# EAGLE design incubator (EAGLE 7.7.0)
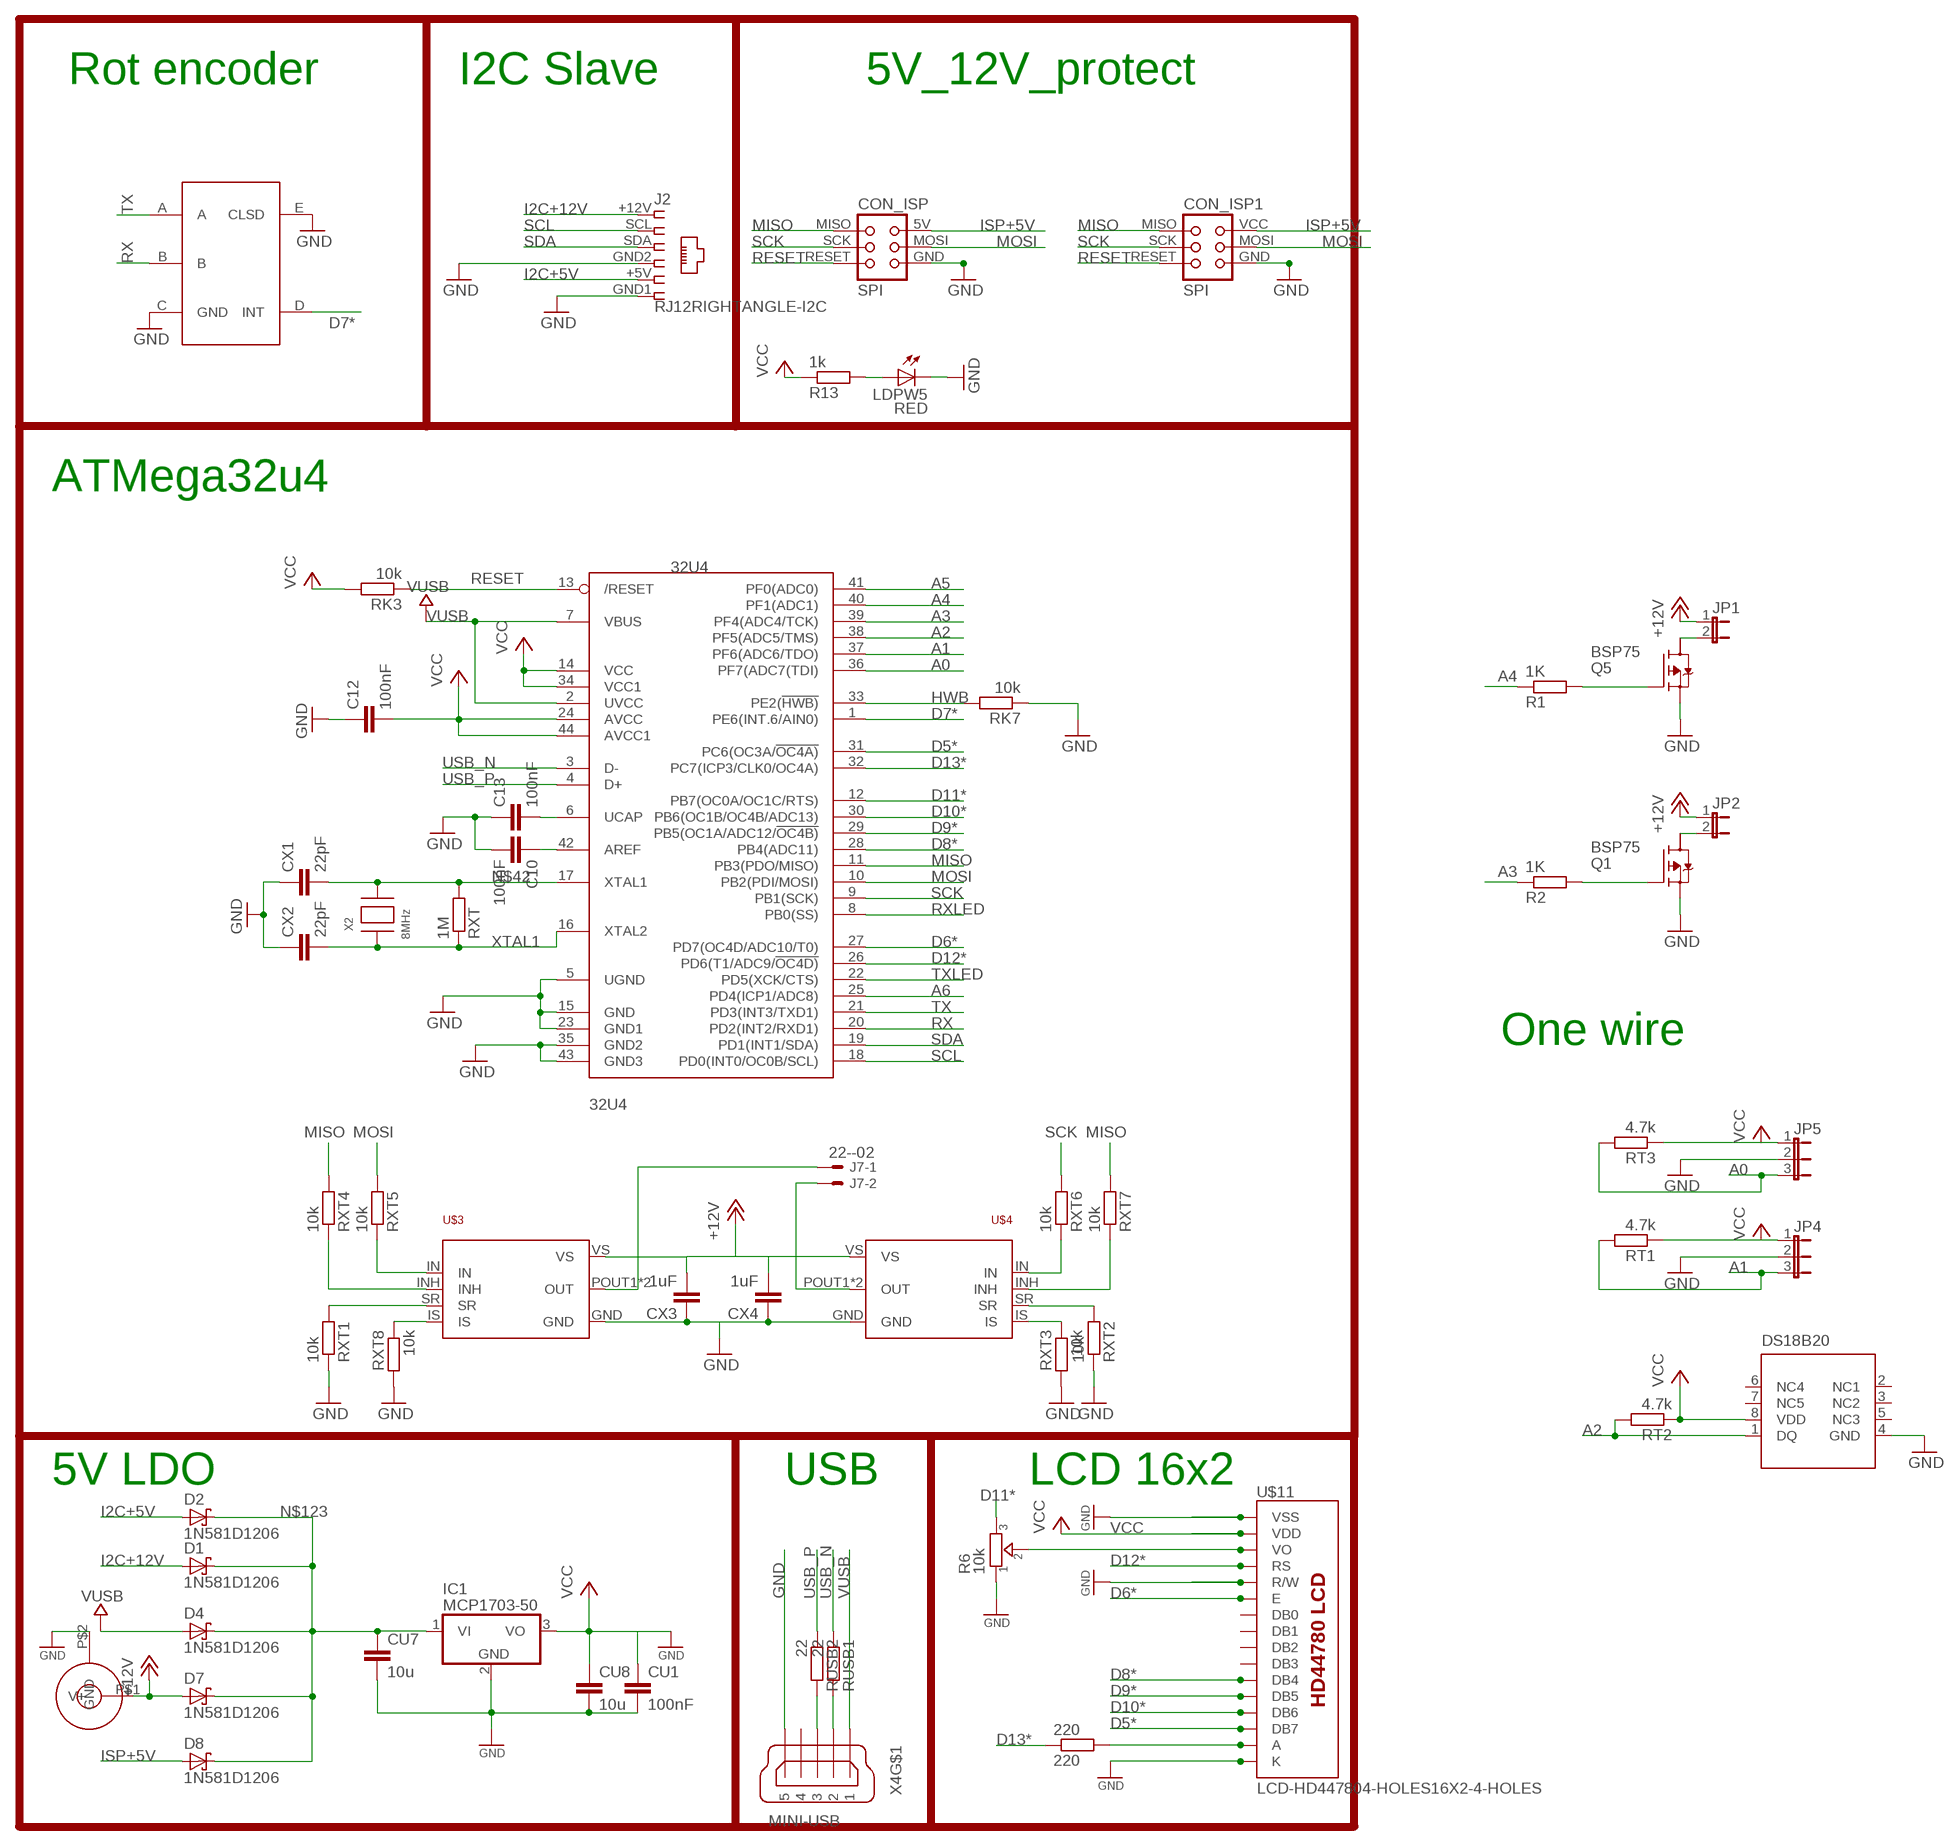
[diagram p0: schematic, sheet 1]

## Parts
32U4  32U4  ATMEGA32U4-AU  [TQFP44]
220  220  R-EU_R0805  [R0805]
C10  100nF  C-EUC0805  [C0805]
C12  100nF  C-EUC0805  [C0805]
C13  100nF  C-EUC0805  [C0805]
CON_ISP  SPI  TINYISPT  [TC2030-MCP-NL]
CON_ISP1  SPI  TINYISP  [TINYISP]
CU1  100nF  C-EUC0805  [C0805]
CU7  10u  C-EUC0805  [C0805]
CU8  10u  C-EUC0805  [C0805]
CX1  22pF  C-EUC0805  [C0805]
CX2  22pF  C-EUC0805  [C0805]
CX3  1uF  C-EUC0805  [C0805]
CX4  1uF  C-EUC0805  [C0805]
D1  1N581D1206  [LED-1206]
D2  1N581D1206  [LED-1206]
D4  1N581D1206  [LED-1206]
D7  1N581D1206  [LED-1206]
D8  1N581D1206  [LED-1206]
IC1  MCP1703-50  MCP1703DB  [SOT223]
J2  RJ12RIGHTANGLE-I2C  [RJ12-RIGHTANGLE-I2C]
J7  22--02  [2-PIN-5.08S]
JP1  JUMPER-2PTH  [1X02]
JP2  JUMPER-2PTH  [1X02]
JP4  JP2E  [JP2]
JP5  JP2E  [JP2]
LDPW5  RED  LEDCHIP-LED0805  [CHIP-LED0805]
POWER  JACK_DC_BARREL  [DC_BARREL]
Q1  BSP75  BSP613P  [PG-SOT-223]
Q5  BSP75  BSP613P  [PG-SOT-223]
R1  1K  R-EU_R0805  [R0805]
R2  1K  R-EU_R0805  [R0805]
R6  10k  TRIMMER-3362P  [TRIMMER_3362P]
R13  1k  R-EU_R0805  [R0805]
RK3  10k  R-EU_M0805  [M0805]
RK7  10k  R-EU_M0805  [M0805]
RT1  4.7k  R-EU_R0805  [R0805]
RT2  4.7k  R-EU_R0805  [R0805]
RT3  4.7k  R-EU_R0805  [R0805]
RUSB1  22  R-EU_M0805  [M0805]
RUSB2  22  R-EU_M0805  [M0805]
RXT  1M  R-EU_R0805  [R0805]
RXT1  10k  R-EU_R0805  [R0805]
RXT2  10k  R-EU_R0805  [R0805]
RXT3  10k  R-EU_R0805  [R0805]
RXT4  10k  R-EU_R0805  [R0805]
RXT5  10k  R-EU_R0805  [R0805]
RXT6  10k  R-EU_R0805  [R0805]
RXT7  10k  R-EU_R0805  [R0805]
RXT8  10k  R-EU_R0805  [R0805]
U$1  EC11E  [EC11E]
U$3  BTS7960  [P-TO-263-7]
U$4  BTS7960  [P-TO-263-7]
U$5  DS18B20  DS18B20SMALL  [MSOP8]
U$11  LCD-HD447804-HOLES16X2-4-HOLES  [LCD-16X2-4HOLES]
X2  8MHz  XTALNX6035  [NX6035]
X4  MINI-USB  MINI-USB-SCHIELD-32005-201  [32005-201]

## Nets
+12V [power]: CX3.2 CX4.2 D7.A JP1.1 JP2.1 POWER.P$1(V+) U$3.VS U$4.VS
A0: 32U4.36(PF7(ADC7(TDI)) JP5.3 RT3.2
A1: 32U4.37(PF6(ADC6/TDO)) JP4.3 RT1.2
A2: 32U4.38(PF5(ADC5/TMS)) RT2.2 U$5.1(DQ)
A3: 32U4.39(PF4(ADC4/TCK)) R2.1
A4: 32U4.40(PF1(ADC1)) R1.1
A5: 32U4.41(PF0(ADC0))
A6: 32U4.25(PD4(ICP1/ADC8))
AREF: 32U4.42(AREF) C10.1
D5*: 32U4.31(PC6(OC3A/!OC4A)) U$11.14(DB7)
D6*: 32U4.27(PD7(OC4D/ADC10/T0)) U$11.6(E)
D7*: 32U4.1(PE6(INT.6/AIN0)) U$1.D(INT)
D8*: 32U4.28(PB4(ADC11)) U$11.11(DB4)
D9*: 32U4.29(PB5(OC1A/ADC12/!OC4B)) U$11.12(DB5)
D10*: 32U4.30(PB6(OC1B/OC4B/ADC13)) U$11.13(DB6)
D11*: 32U4.12(PB7(OC0A/OC1C/RTS)) R6.3
D12*: 32U4.26(PD6(T1/ADC9/!OC4D)) U$11.4(RS)
D13*: 32U4.32(PC7(ICP3/CLK0/OC4A)) 220.1
GND [power]: 32U4.5(UGND) 32U4.15(GND) 32U4.23(GND1) 32U4.35(GND2) 32U4.43(GND3) C10.2 C12.1 C13.1 CON_ISP1.GND CON_ISP.GND CU1.2 CU7.2 CU8.2 CX1.1 CX2.1 CX3.1 CX4.1 IC1.2(GND) J2.GND1 J2.GND2 JP4.2 JP5.2 LDPW5.C POWER.P$2(GND) Q1.3(S) Q5.3(S) R6.1 RK7.1 RXT1.1 RXT2.1 RXT3.2 RXT8.2 U$1.C(GND) U$1.E(CLSD) U$3.GND U$4.GND U$5.4(GND) U$11.1(VSS) U$11.5(R/W) U$11.16(K) X4.5
HWB: 32U4.33(PE2(!HWB)) RK7.2
I2C+5V: D2.A J2.+5V
I2C+12V [power]: D1.A J2.+12V
ISP+5V: CON_ISP1.VCC CON_ISP.5V(VCC) D8.A
MISO: 32U4.11(PB3(PDO/MISO)) CON_ISP1.MISO CON_ISP.MISO RXT4.2 RXT7.2
MOSI: 32U4.10(PB2(PDI/MOSI)) CON_ISP1.MOSI CON_ISP.MOSI RXT5.2
N$1: 32U4.6(UCAP) C13.2
N$2: R6.2 U$11.3(VO)
N$4: RXT5.1 U$3.IN
N$5: RXT6.1 U$4.IN
N$6: RXT4.1 U$3.INH
N$7: RXT7.1 U$4.INH
N$8: RXT3.1 U$4.IS
N$9: Q5.1(G) R1.2
N$10: RXT2.2 U$4.SR
N$11: 220.2 U$11.15(A)
N$12: LDPW5.A R13.2
N$13: RXT1.2 U$3.SR
N$14: RXT8.1 U$3.IS
N$19: J7.1 U$3.POUT1(OUT) U$3.POUT2(OUT)
N$20: Q1.1(G) R2.2
N$21: JP1.2 Q5.2(D)
N$22: J7.2 U$4.POUT1(OUT) U$4.POUT2(OUT)
N$23: JP2.2 Q1.2(D)
N$42: 32U4.17(XTAL1) CX1.2 RXT.2 X2.P$2
N$123: CU7.1 D1.C D2.C D4.C D7.C D8.C IC1.1(VI)
RESET: 32U4.13(/RESET) CON_ISP1.RESET CON_ISP.RESET RK3.1
RX: 32U4.20(PD2(INT2/RXD1)) U$1.B
RXLED: 32U4.8(PB0(SS))
SCK: 32U4.9(PB1(SCK)) CON_ISP1.SCK CON_ISP.SCK RXT6.2
SCL: 32U4.18(PD0(INT0/OC0B/SCL)) J2.SCL
SDA: 32U4.19(PD1(INT1/SDA)) J2.SDA
TX: 32U4.21(PD3(INT3/TXD1)) U$1.A
TXLED: 32U4.22(PD5(XCK/CTS))
USB_N: 32U4.3(D-) RUSB1.1
USB_P: 32U4.4(D+) RUSB2.1
USBC_N: RUSB1.2 X4.2
USBC_P: RUSB2.2 X4.3
VCC: 32U4.14(VCC) 32U4.24(AVCC) 32U4.34(VCC1) 32U4.44(AVCC1) C12.2 CU1.1 CU8.1 IC1.3(VO) JP4.1 JP5.1 R13.1 RK3.2 RT1.1 RT2.1 RT3.1 U$5.8(VDD) U$11.2(VDD) ; supply symbol labelled GND
VUSB: 32U4.2(UVCC) 32U4.7(VBUS) D4.A X4.1
XTAL1: 32U4.16(XTAL2) CX2.2 RXT.1 X2.P$1
Unconnected: Q1.4(D) Q5.4(D) U$5.2(NC1) U$5.3(NC2) U$5.5(NC3) U$5.6(NC4) U$5.7(NC5) U$11.7(DB0) U$11.8(DB1) U$11.9(DB2) U$11.10(DB3) X4.4 X4.M1(S:S1) X4.M2(S:S2) X4.M3(S:S3) X4.M4(S:S4)

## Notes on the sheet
- Rot encoder | I2C Slave | 5V_12V_protect
- ATMega32u4
- One wire
- 5V LDO | USB | LCD 16x2

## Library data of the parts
32U4 = adafruit:ATMEGA32U4: http://www.ladyada.net/library/eagle
220 R1 R2 RXT RXT1-RXT8 = rcl:R-EU_: RESISTOR, European symbol
C10 C12 C13 CU1 CU7 CU8 CX1-CX4 = rcl:C-EU: CAPACITOR, European symbol
CON_ISP = lpatiny:TINYISP: CONNECTOR
CON_ISP1 = lpatiny:TINYISP: CONNECTOR; OC_FARNELL: unknown; OC_NEWARK: unknown
D1 D2 D4 D7 D8 = lpatiny:1N581*: 1.0A SCHOTTKY BARRIER RECTIFIER
IC1 = linear:MCP1703: 250 mA, 16V, Low Quiescent Current LDO Regulator Source: http://ww1.microchip.com/downloads/en/DeviceDoc/22049b.pdf
J2 = lpatiny:RJ12: CORCOM Modular RJ Jacks No Shield Source: www.tycoelectronics.com .. ENG_DS_1654001_1099_RJ_L_0507.pdf
J7 = lpatiny:22-?-02: CONNECTOR
JP1 JP2 = SparkFun:JUMPER-2: Jumper
JP4 JP5 = jumper:JP2E: JUMPER
LDPW5 = adafruit:LED: LED
POWER = lpatiny:JACK_DC_BARREL
Q1 Q5 = infineon:BSP613P: SIPMOS (R) Small-Signal-Transistor P-Channel (2 Drain) Source: http://www.infineon.com/dgdl/BSP613P_Rev2.4.pdf; OC_FARNELL: unknown; OC_NEWARK: unknown
R6 = dp_devices:TRIMMER: Trimmer resistor
R13 RK3 RK7 RT1-RT3 RUSB1 RUSB2 = resistor:R-EU_: RESISTOR, European symbol
U$1 = lpatiny:EC11E: ALPS Rotary encoder
U$3 U$4 = BTS7960:BTS7960; AVAILABILITY: Warning; DESCRIPTION: Half Bridge Motor Driver 7-Pin%286%2BTab%29 TO-263; MF: Infineon; MP: BTS7960B; PACKAGE: TO-263 Infineon; PRICE: 4.95 USD
U$5 = lpatiny:DS18B20
U$11 = HD44780LCD:LCD-HD44780
X2 = lpatiny:XTAL: Low cost SMT crystals, no capacitors included
X4 = con-cypressindustries:MINI-USB-SCHIELD-: MINI USB-B Conector Source: www.cypressindustries.com; OC_FARNELL: unknown; OC_NEWARK: unknown

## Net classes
0 default: width 0.203 mm, clearance 0.25 mm
1 power: width 0.203 mm, drill 0.305 mm, clearance 0.25 mm
2 VIN: width 0.406 mm, clearance 0.25 mm
3 fine: width 0.406 mm, clearance 0.25 mm
4 aref: width 0.406 mm, clearance 0.25 mm

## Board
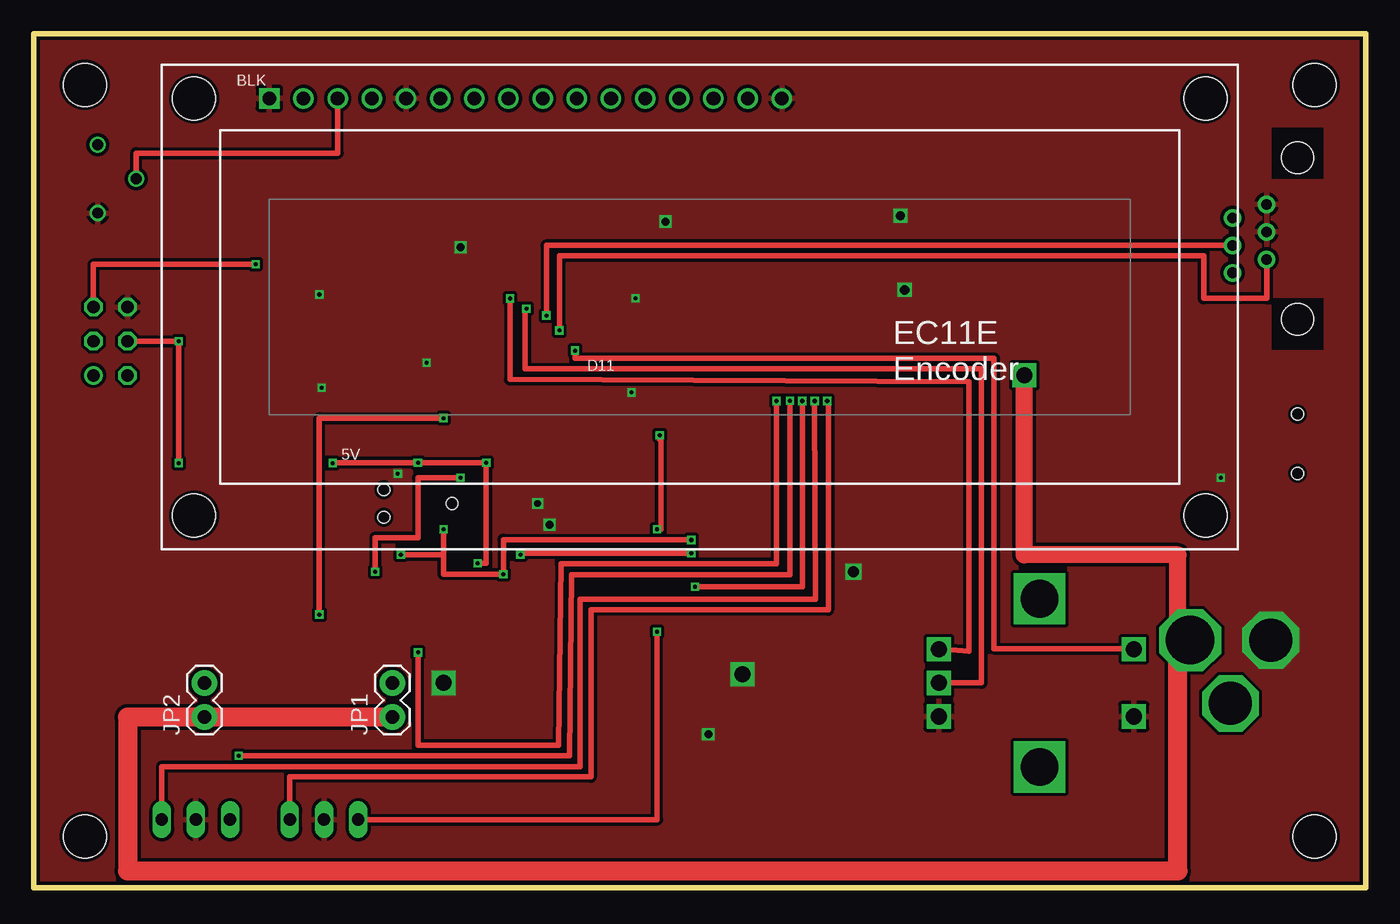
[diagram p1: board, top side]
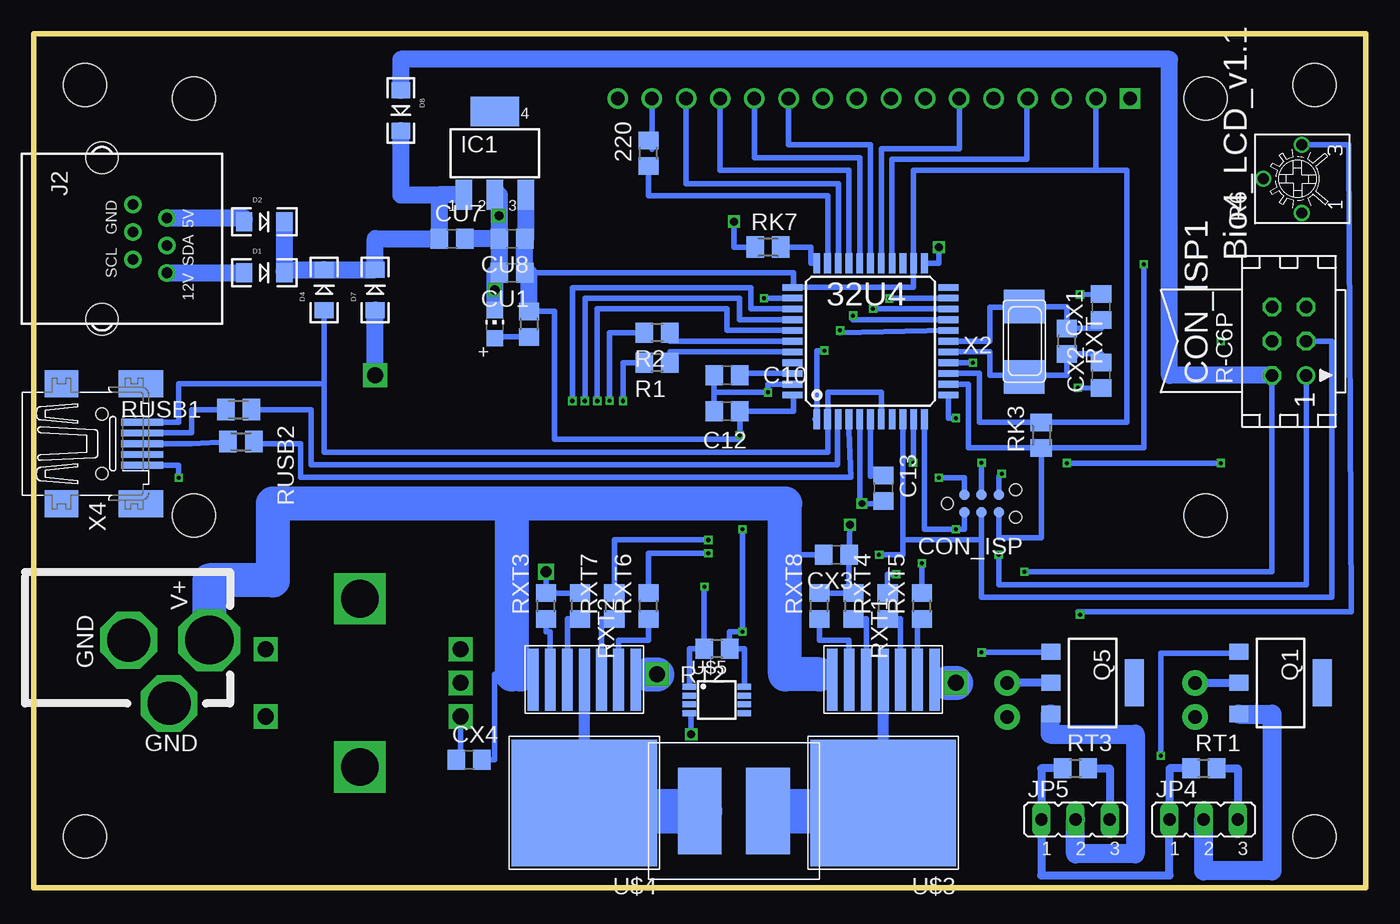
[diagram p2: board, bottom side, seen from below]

Size 99.06 x 63.5 mm. Coordinates in mm from the lower left corner, seen from the top.
Outline: 0,63.5 0,0 99.06,0 99.06,63.5 0,63.5
Copper layers (1*2*15*16): Top 0.035mm / dielectric 0.2mm / layer 2 0.0175mm / dielectric 1.1mm / layer 15 0.0175mm / dielectric 0.2mm / Bottom 0.035mm
Design rules "SeeedStudio_DRU_no_angle_20130527": minimum track width 6mil, minimum drill 12mil, track to track 6mil, track to pad 6mil, pad to pad 6mil, via to via 6mil, smd to smd 0mil, copper to edge 10mil, drill to drill 10mil, minimum pad ring 6mil, minimum via ring 6mil, stop-mask expansion 2mil, vias tented up to drill 25mil, thermal gap 10mil
Holes 3.2 mm at 3.81,59.69 3.81,3.81 95.25,59.69 95.25,3.81

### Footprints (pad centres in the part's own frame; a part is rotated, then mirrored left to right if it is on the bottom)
TQFP44 = smd 1.5 x 0.5: 1 -5.8,4; 2 -5.8,3.2; 3 -5.8,2.4; 4 -5.8,1.6; 5 -5.8,0.8; 6 -5.8,0; 7 -5.8,-0.8; 8 -5.8,-1.6; 9 -5.8,-2.4; 10 -5.8,-3.2; 11 -5.8,-4; 23 5.8,-4; 24 5.8,-3.2; 25 5.8,-2.4; 26 5.8,-1.6; 27 5.8,-0.8; 28 5.8,0; 29 5.8,0.8; 30 5.8,1.6; 31 5.8,2.4; 32 5.8,3.2; 33 5.8,4 | smd 0.5 x 1.5: 12 -4,-5.8; 13 -3.2,-5.8; 14 -2.4,-5.8; 15 -1.6,-5.8; 16 -0.8,-5.8; 17 0,-5.8; 18 0.8,-5.8; 19 1.6,-5.8; 20 2.4,-5.8; 21 3.2,-5.8; 22 4,-5.8; 34 4,5.8; 35 3.2,5.8; 36 2.4,5.8; 37 1.6,5.8; 38 0.8,5.8; 39 0,5.8; 40 -0.8,5.8; 41 -1.6,5.8; 42 -2.4,5.8; 43 -3.2,5.8; 44 -4,5.8
R0805 = smd 1.3 x 1.5: 1 -0.95,0; 2 0.95,0
C0805 = smd 1.3 x 1.5: 1 -0.95,0; 2 0.95,0
TC2030-MCP-NL = smd 0.787 x 0.787: 5V 1.27,0.635; GND 3.81,0.635; MISO 1.27,-0.635; MOSI 2.54,0.635; RESET 3.81,-0.635; SCK 2.54,-0.635 | hole 0.889: 0,0; 5.08,-1.016; 5.08,1.016
TINYISP = drill 0.914 octagon: GND 2.54,1.27; MOSI 0,1.27; RESET 2.54,-1.27; SCK 0,-1.27; VCC -2.54,1.27 | drill 0.914: MISO -2.54,-1.27
LED-1206 = smd 1.2 x 1.4: A -1.5,0; C 1.5,0
SOT223 = smd 1.219 x 2.235: 1 -2.311,-3.099; 2 0,-3.099; 3 2.311,-3.099 | smd 3.6 x 2.2: 4 0,3.099
RJ12-RIGHTANGLE-I2C = drill 0.8 pad 1.3: +5V -1.54,4.84; +12V 2.54,4.84; GND1 -2.54,2.3; GND2 -0.5,2.3; SCL 1.54,2.3; SDA 0.5,4.84 | hole 2.36: -6,0; 6,0
2-PIN-5.08S = smd 3.251 x 6.452: 1 -2.54,0; 2 2.54,0
1X02 = drill 1.016 pad 1.88: 1 0,0; 2 2.54,0
JP2 = drill 0.914 long: 1 -2.54,0; 2 0,0; 3 2.54,0
CHIP-LED0805 = smd 1.2 x 1.2: A 0,-1.05; C 0,1.05
DC_BARREL = drill 3.6 pad 4.5 octagon: P$1 0,13.7 | drill 3.2 pad 4.064 octagon: P$2 0,7.7; P$3 4.7,10.7
PG-SOT-223 = smd 1.2 x 1.4: 1 -2.311,-3.099; 2 0,-3.099; 3 2.311,-3.099 | smd 3.5 x 1.4: 4 0,3.099
TRIMMER_3362P = drill 0.8: 1 -2.54,-0.31; 2 0,2.54; 3 2.54,-0.31
M0805 = smd 1.3 x 1.6: 1 -0.95,0; 2 0.95,0
EC11E = drill 1.2 square: A -2.5,0; B 0,0; C 2.5,0; D -2.5,14.5; E 2.5,14.5 | drill 2.8 square: P$1 6.25,7.5; P$2 -6.25,7.5
P-TO-263-7 = smd 0.8 x 4.6: GND 1.59,2.3; IN 2.86,2.3; INH 4.13,2.3; IS 7.94,2.3; POUT2 5.4,2.3; SR 6.67,2.3; VS 9.21,2.3 | smd 10.8 x 9.4: POUT1 5.4,11.45
MSOP8 = smd 0.45 x 1: 1 -0.975,-2.05; 2 -0.325,-2.05; 3 0.325,-2.05; 4 0.975,-2.05; 5 0.975,2.05; 6 0.325,2.05; 7 -0.325,2.05; 8 -0.975,2.05
LCD-16X2-4HOLES = drill 1.016 square: 1 -32,15.5 | drill 1.016: 2 -29.46,15.5; 3 -26.92,15.5; 4 -24.38,15.5; 5 -21.84,15.5; 6 -19.3,15.5; 7 -16.76,15.5; 8 -14.22,15.5; 9 -11.68,15.5; 10 -9.14,15.5; 11 -6.6,15.5; 12 -4.06,15.5; 13 -1.52,15.5; 14 1.02,15.5; 15 3.56,15.5; 16 6.1,15.5 | hole 3.2: -37.6,15.5; -37.6,-15.5; 37.6,-15.5; 37.6,15.5
NX6035 = smd 2.5 x 3: P$1 2.665,0; P$2 -2.565,0
32005-201 = smd 3.1 x 0.5: 1 3,1.6; 2 3,0.8; 3 3,0; 4 3,-0.8; 5 3,-1.6 | smd 2.5 x 2: M1 -3,-4.45; M2 -3,4.45 | smd 3.3 x 2: M3 2.9,4.45; M4 2.9,-4.45 | hole 0.9: 0,2.2; 0,-2.2

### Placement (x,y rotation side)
32U4  36.83,40.64 90 bottom
220  53.34,54.61 90 bottom
C10  47.5,38.1 180 bottom
C12  47.5,35.44 0 bottom
C13  35.88,29.72 90 bottom
CON_ISP  31.11,28.57 0 bottom
CON_ISP1  5.71,40.64 90 bottom
CU1  63.5,45.72 180 bottom
CU7  67.94,48.26 0 bottom
CU8  63.5,48.26 180 bottom
CX1  19.68,43.18 270 bottom
CX2  19.68,38.1 90 bottom
CX3  39.37,24.77 180 bottom
CX4  66.67,9.53 0 bottom
D1  81.92,45.72 0 bottom
D2  81.92,49.53 0 bottom
D4  77.47,44.45 90 bottom
D7  73.66,44.45 90 bottom
D8  71.75,57.78 270 bottom
IC1  64.77,54.61 0 bottom
J2  93.98,48.26 270 bottom
J7  46.99,5.71 180 bottom
JP1  26.67,12.7 90 top
JP2  12.7,12.7 90 top
JP4  12.06,5.08 0 bottom
JP5  21.59,5.08 0 bottom
LDPW5  64.77,41.91 0 bottom
POWER  99.69,18.41 270 bottom
Q1  6.35,15.24 270 bottom
Q5  20.32,15.24 270 bottom
R1  52.7,39.03 180 bottom
R2  52.7,41.27 180 bottom
R6  5.08,52.7 90 bottom
R13  62.23,41.91 270 bottom
RK3  24.13,33.66 90 bottom
RK7  44.45,47.62 0 bottom
RT1  12.06,8.89 0 bottom
RT2  48.26,17.78 180 bottom
RT3  21.59,8.89 0 bottom
RUSB1  83.82,35.56 180 bottom
RUSB2  83.65,33.17 180 bottom
RXT  22.23,40.64 90 bottom
RXT1  38.1,20.95 270 bottom
RXT2  58.42,20.95 270 bottom
RXT3  60.96,20.95 90 bottom
RXT4  35.56,20.95 90 bottom
RXT5  33.02,20.95 90 bottom
RXT6  53.34,20.95 90 bottom
RXT7  55.88,20.95 90 bottom
RXT8  40.64,20.95 90 bottom
U$1  67.31,15.24 270 top
U$3  30.48,17.78 180 bottom
U$4  52.7,17.78 180 bottom
U$5  48.26,13.97 270 bottom
U$11  49.53,43.18 0 top
X2  25.4,40.64 270 bottom
X4  93.98,33.02 0 bottom

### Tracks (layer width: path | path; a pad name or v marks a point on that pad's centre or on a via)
+12V  (via drill 1.2)
  Top 1.27: 85.09,18.41 85.09,24.77 73.66,24.77 v73.66,38.1
  Top 1.422: JP1.1 JP2.1 6.99,12.7 6.99,1.27 85.09,1.27 85.09,18.41 POWER.P$1
  Bottom 0.406: CX4.2 64.77,9.53 64.77,15.88 63.5,15.88 | CX3.2 43.18,24.77
  Bottom 0.813: U$3.VS 40.64,15.48 40.64,15.88 | U$4.VS 62.87,15.48 62.87,15.88
  Bottom 1.27: v73.66,38.1 D7.A
  Bottom 2.54: 40.64,15.88 43.18,15.88 43.18,24.77 43.18,28.57 63.5,28.57 | 63.5,28.57 81.28,28.57 81.28,22.86 86,22.86 POWER.P$1 | 62.87,15.88 63.5,15.88 63.5,28.57
A0  (via drill 0.3)
  Top 0.406: v59,36.2 59.1,36.2 59.1,20.68 41.45,20.68 41.45,8.26 19.05,8.26 JP5.3
  Bottom 0.406: 32U4.36 45.72,43.04 45.72,44.62 59,44.62 v59,36.2
  Bottom 0.61: RT3.2 19.05,8.89 JP5.3
A1  (via drill 0.3)
  Top 0.406: v58.08,36.2 58.13,21.47 40.64,21.47 40.64,9.01 9.53,9.01 JP4.3
  Bottom 0.406: 32U4.37 46.56,42.24 46.56,43.81 58.08,43.81 v58.08,36.2
  Bottom 0.61: RT1.2 9.53,8.89 JP4.3
A2  (via drill 0.3)
  Top 0.406: v57.15,36.2 57.15,22.4 v49.19,22.4
  Bottom 0.406: U$5.1 50.31,17.78 RT2.2 49.21,22.23 v49.19,22.4 | 32U4.38 47.49,41.44 47.49,43.03 57.15,43.03 v57.15,36.2
A3
  Bottom 0.406: 32U4.39 51.76,40.64 R2.1
A4
  Bottom 0.406: 42.63,39.88 32U4.40 51.76,39.84 R1.1
AREF
  Bottom 0.406: 32U4.42 46.55,38.24 C10.1
D5*
  Bottom 0.406: 39.24,46.44 32U4.31 39.23,52.34 50.55,52.34 U$11.14
D6*
  Bottom 0.406: 32U4.27 36.03,54.93 30.23,54.93 U$11.6
D7*  (via drill 0.3)
  Top 0.406: v40.26,39.94 40.26,39.37 71.41,39.37 71.41,17.78 81.81,17.78 U$1.D
  Bottom 0.406: 40.96,34.84 32U4.1 40.83,39.94 v40.26,39.94
D8*
  Bottom 0.406: 32U4.28 36.83,55.24 42.93,55.24 U$11.11
D9*
  Bottom 0.406: 32U4.29 37.63,54.29 45.47,54.29 U$11.12
D10*
  Bottom 0.406: 32U4.30 38.43,53.34 48.01,53.34 U$11.13
D11*  (via drill 0.3)
  Top 0.406: v21.25,20.32 21.25,34.92 v30.48,34.92
  Bottom 0.406: R6.3 1.27,55.24 1.1,20.54 21.42,20.54 v21.25,20.32 | v30.48,34.92 31.03,34.92 32U4.12
D12*
  Bottom 0.406: U$11.4 25.2,58.68 25.2,54.18 35.23,54.18 32U4.26
D13*
  Bottom 0.406: 32U4.32 40.01,46.44 40.01,51.44 53.34,51.44 220.1
GND  (via drill 0.3, 0.5 pad 0.61, 0.6, 0.7, 0.8, 1.2)
  Bottom 0.406: 32U4.43 44.45,37.44 v44.45,36.83 48.45,36.83 C10.2 C12.1 | 32U4.5 37.63,28.57 v37.47,28.57 35.88,28.57 C13.1 | 64.77,48.26 CU8.2 | CU1.2 64.77,45.72 | 91.68,48.74 J2.GND2 | X4.5 88.27,31.42 v88.27,30.48 | v44.77,43.84 32U4.35 | CX1.1 v21.25,44.11 | 32U4.15 v29.22,39.04 | v29.22,39.04 | 32.85,46.44 32U4.23 31.75,46.44 v31.75,47.62 | CON_ISP.GND 27.3,30.56 v27.08,30.79 | RK7.1 46.99,47.62 v46.99,49.53 | CX2.1 v21.42,37.17 | RXT8.2 RXT1.1 38.42,21.91 CX3.1 v38.37,26.99 | U$1.C 67.31,9.53 CX4.1 | U$5.4 arc90 50.16,12.85 v50.16,11.43 | RXT2.1 RXT3.2 v60.96,23.5
  Bottom 0.813: U$4.GND 53.34,15.48 53.34,15.88 | U$3.GND 31.75,15.48 31.11,15.24
  Bottom 1.27: IC1.2 64.45,51.51 v64.45,49.97 CU8.2 | CU8.2 CU7.2 | CU8.2 CU1.2 | LDPW5.C v64.77,44.45 64.77,45.72
  Bottom 1.422: Q1.3 6.99,12.93 6.99,1.27 12.06,1.27 JP4.2 | Q5.3 23.5,12.93 23.5,11.43 17.14,11.43 17.14,2.54 21.59,2.54 JP5.2
  Bottom 2.54: 53.34,15.88 v52.7,15.88 | 31.11,15.24 v30.48,15.24
  pour Top: 0,63.5 0,0 99.06,0 99.06,63.5
HWB
  Bottom 0.406: 32U4.33 41.27,46.44 41.27,47.62 RK7.2
I2C+5V
  Bottom 1.27: J2.+5V 83.42,49.8 D2.A
I2C+12V
  Bottom 1.27: J2.+12V D1.A
ISP+5V  (via drill 0.3)
  Top 0.406: v31.75,30.48 28.57,30.48 28.57,26.04 25.4,26.04 v25.4,23.5
  Bottom 0.406: CON_ISP.5V 29.84,30.48 v31.75,30.48 | v25.4,23.5 6.99,23.5 CON_ISP1.VCC
  Bottom 1.27: CON_ISP1.VCC 14.61,38.1 14.61,61.59 71.75,61.59 D8.A
MISO  (via drill 0.3)
  Top 0.406: v27.3,24.77 30.48,24.77 v30.48,26.67 30.48,23.32 v34.92,23.32 34.92,25.89 48.9,25.89 v48.9,25.86
  Bottom 0.406: CON_ISP.MISO 29.84,26.67 v30.48,26.67 32.83,26.67 32U4.11 | CON_ISP1.MISO 4.45,22.53 27.3,22.53 v27.3,24.77 | RXT7.2 55.88,25.86 v48.9,25.86 | v34.92,23.32 35.56,23.32 RXT4.2
MOSI  (via drill 0.3)
  Top 0.406: CON_ISP1.MOSI v10.79,40.64 v10.79,31.58 | v22.23,31.58 22.23,31.61 v28.57,31.61 v33.66,31.61 33.66,24.13 v33.02,24.13
  Bottom 0.406: CON_ISP.MOSI v28.57,31.61 | v22.23,31.58 v10.79,31.58 | 32U4.10 33.66,34.84 v33.66,31.61 | v33.02,24.13 RXT5.2
N$1
  Bottom 0.406: C13.2 36.83,30.61 32U4.6
N$2
  Top 0.406: R6.2 7.62,54.61 22.61,54.61 U$11.3
  Bottom 0.406: U$11.3
N$4
  Bottom 0.406: RXT5.1 33.34,20 U$3.IN
N$5
  Bottom 0.406: RXT6.1 53.34,18.41 55.56,18.41 U$4.IN
N$6
  Bottom 0.406: RXT4.1 34.61,20 U$3.INH
N$7
  Bottom 0.406: RXT7.1 56.84,20 U$4.INH
N$8
  Bottom 0.406: RXT3.1 60.96,19.05 60.65,19.05 U$4.IS
N$9  (via drill 0.3)
  Top 0.406: v55.24,36.2 55.24,24.08 39.2,24.08 39.03,10.62 28.57,10.62 v28.57,17.51
  Bottom 0.406: R1.2 55.24,39.03 v55.24,36.2 | v28.57,17.51 23.42,17.51 Q5.1
N$10
  Bottom 0.406: RXT2.2 59.38,20 U$4.SR
N$11
  Bottom 0.406: U$11.15 53.09,54.92 220.2
N$12
  Bottom 0.406: R13.2 64.77,40.96 LDPW5.A
N$13
  Bottom 0.406: RXT1.2 37.15,20 U$3.SR
N$14
  Bottom 0.406: RXT8.1 40.64,18.41 38.42,18.41 U$3.IS
N$19
  Bottom 0.813: U$3.POUT1 U$3.POUT2
  Bottom 3.302: J7.1 35.88,5.71 U$3.POUT1
N$20  (via drill 0.3)
  Top 0.406: v56.24,36.21 56.24,23.27 40.01,23.27 39.83,9.82 v15.24,9.82
  Bottom 0.406: R2.2 56.24,41.27 v56.24,36.21 | v15.24,9.82 15.24,17.44 9.45,17.44 Q1.1
N$21
  Bottom 0.61: Q5.2 JP1.2
N$22
  Bottom 0.813: U$4.POUT1 U$4.POUT2
  Bottom 3.302: J7.2 58.1,5.71 U$4.POUT1
N$23
  Bottom 0.61: JP2.2 Q1.2
N$42
  Bottom 0.406: 32U4.17 27.94,40.64 27.94,43.18 25.4,43.18 X2.P$2 22.23,43.2 RXT.2 19.68,41.59 CX1.2
N$123
  Bottom 0.406: CU7.1 69.22,48.26
  Bottom 1.27: D8.C 71.75,51.51 68.89,51.51 | D2.C D1.C 80.42,45.95 D4.C D7.C 73.66,48.26 CU7.1 68.89,51.51 | IC1.1 68.89,51.51
RESET  (via drill 0.3)
  Top 0.406: v16.51,46.35 4.45,46.35 CON_ISP1.RESET
  Bottom 0.406: 32U4.13 29.54,37.44 29.54,32.7 RK3.1 | CON_ISP.RESET 27.3,26.04 24.13,26.04 RK3.1 | RK3.1 16.51,32.7 v16.51,46.35
RX  (via drill 0.3)
  Top 0.406: v36.64,43.05 36.52,43.05 36.52,38.59 70.48,38.59 70.48,15.24 U$1.B
  Bottom 0.406: 32U4.20 34.1,43.04 v36.64,43.05
SCK  (via drill 0.3)
  Top 0.406: v48.9,24.89 36.2,24.89 v36.2,24.77
  Bottom 0.406: CON_ISP.SCK 28.57,25.87 | 28.57,25.87 34.43,25.87 | 34.43,25.87 32U4.9 | CON_ISP1.SCK 2.54,40.64 2.54,21.59 28.57,21.59 28.57,25.87 | RXT6.2 53.34,24.89 v48.9,24.89 | v36.2,24.77 34.43,24.77 34.43,25.87
SCL  (via drill 0.3)
  Top 0.406: v39.09,41.44 39.09,46.99 87,46.99 87,43.81 91.68,43.81 J2.SCL
  Bottom 0.406: v39.09,41.44 39.09,41.27 32U4.18
SDA  (via drill 0.3)
  Top 0.406: J2.SDA 38.12,47.76 v38.12,42.55
  Bottom 0.406: v38.12,42.55 38.15,42.24 32U4.19
TX  (via drill 0.3)
  Top 0.406: v35.42,43.81 35.42,37.81 69.56,37.64 69.56,17.61 67.31,17.78 U$1.A
  Bottom 0.406: 32U4.21 v35.42,43.81
USB_N
  Bottom 0.406: 32U4.3 39.29,34.84 39.29,31.46 52.7,31.46 52.7,31.45 78.42,31.45 78.42,35.56 RUSB1.1
USB_P
  Bottom 0.406: 32U4.4 38.47,34.84 38.3,30.53 79.2,30.53 79.2,33 82.7,33 RUSB2.1
USBC_N
  Bottom 0.406: X4.2 87.3,33.82 87.3,35.56 RUSB1.2
USBC_P
  Bottom 0.406: X4.3 87.3,33.02 87.3,33 RUSB2.2
VCC  (via drill 0.3)
  Top 0.406: JP5.1 46.35,5.08 v46.35,19.05 | v46.35,26.67 46.63,26.67 46.63,33.36 46.55,33.36 v46.55,33.66
  Bottom 0.406: 32U4.44 42.55,36.64 42.55,35.44 C12.2 v46.55,33.66 46.55,33.36 60.33,33.36 60.33,42.86 R13.1 | 32U4.14 28.74,38.24 28.74,34.6 RK3.2 17.78,34.6 17.78,53.34 20.07,53.34 | U$5.8 46.21,17.78 RT2.1 47.31,19.05 v46.35,19.05 v46.35,26.67 | CU1.1 42.55,45.72 42.55,44.64 32U4.34 33.66,44.64 33.66,46.44 | 32U4.24 33.66,46.44 | U$11.2 20.07,53.34 | 20.07,53.34 33.66,53.34 33.66,46.44
  Bottom 0.61: RT1.1 14.61,8.89 JP4.1 14.61,0.93 24.13,0.93 JP5.1 24.13,8.89 RT3.1
  Bottom 0.813: IC1.3 62.23,51.51
  Bottom 1.27: R13.1 62.23,45.72 CU1.1 CU8.1 62.46,48.26 IC1.3
VUSB
  Bottom 0.406: 40.01,34.84 40.01,36.83 36.03,36.83 32U4.7 | 32U4.2 40.01,34.84 | 40.01,34.84 40.01,32.38 77.47,32.38 77.47,37.47 | 77.47,37.47 88.27,37.47 88.27,34.62 X4.1 | D4.A 77.47,37.47
XTAL1
  Bottom 0.406: RXT.1 22.23,38.1 25.4,38.1 | 25.4,38.1 X2.P$1 | 25.4,38.1 27.94,38.1 27.94,39.84 32U4.16 | 21.59,39.5 RXT.1 | CX2.2 19.68,39.69 RXT.1

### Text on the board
tNames: 1 | BLK | D11 | EC11E / Encoder | 5V
bNames: Bio4_LCD_v1.1
tValues: Incubator v1.0.0
bValues: Incubator v1.0.0

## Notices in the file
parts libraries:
lpatiny: ©2009 ROFA.cz - modified and updated by Robert Darlington ‹rdarlington@gmail.com›
SparkFun: Licensing: CC v3.0 Share-Alike You are welcome to use this library for commercial purposes.
